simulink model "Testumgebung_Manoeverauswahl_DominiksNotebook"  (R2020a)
settings: Solver=ode4  StartTime=0.0  StopTime=30.0  FixedStep=0.01  RelTol=1e-3
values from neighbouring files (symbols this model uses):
  c = [0;0]    [Testskript_Manoeverauswahl.m]

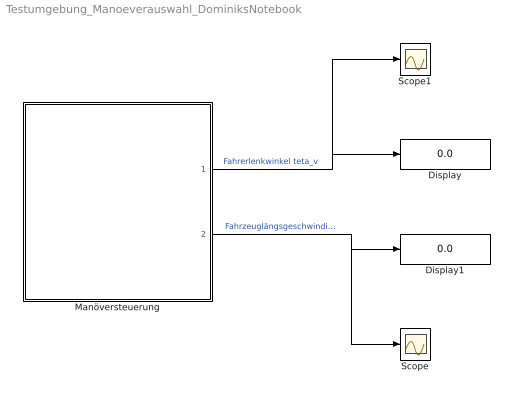
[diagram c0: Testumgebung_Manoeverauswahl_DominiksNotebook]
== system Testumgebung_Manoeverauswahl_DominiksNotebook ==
  Display : Display
  Display1 : Display
  Manöversteuerung : Subsystem
  Scope : Scope
  Scope1 : Scope
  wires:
  Manöversteuerung/2(Fahrzeuglängsgeschwindigkeit KvCx) -> Scope/1, Display1/1  "Fahrzeuglängsgeschwindigkeit KvCx"
  Manöversteuerung/1(Fahrerlenkwinkel teta_v) -> Scope1/1, Display/1  "Fahrerlenkwinkel teta_v"

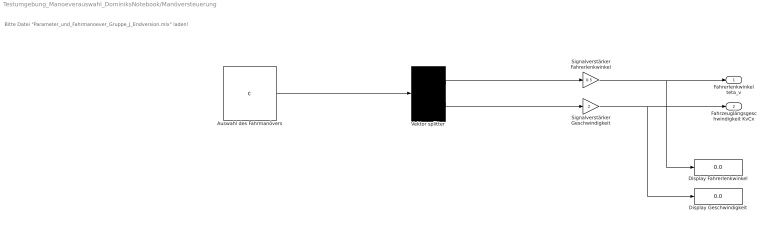
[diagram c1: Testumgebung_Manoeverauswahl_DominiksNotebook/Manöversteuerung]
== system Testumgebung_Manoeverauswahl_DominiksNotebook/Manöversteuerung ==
  note: Bitte Datei "Parameter_und_Fahrmanoever_Gruppe_J_Endversion.mlx" laden!
  Auswahl des Fahrmanövers : Constant  Value=c
  Display Fahrerlenkwinkel : Display
  Display Geschwindigkeit : Display
  Signalverstärker Fahrerlenkwinkel : Gain  Gain=0.5
  Signalverstärker Geschwindigkeit : Gain  Gain=2
  Vektor splitter : Demux  Outputs=2
  Fahrerlenkwinkel teta_v : Outport
  Fahrzeuglängsgeschwindigkeit KvCx : Outport  Port=2
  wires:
  Vektor splitter/1 -> Signalverstärker Fahrerlenkwinkel/1
  Vektor splitter/2 -> Signalverstärker Geschwindigkeit/1
  Signalverstärker Geschwindigkeit/1 -> Fahrzeuglängsgeschwindigkeit KvCx/1, Display Geschwindigkeit/1
  Signalverstärker Fahrerlenkwinkel/1 -> Fahrerlenkwinkel teta_v/1, Display Fahrerlenkwinkel/1
  Auswahl des Fahrmanövers/1 -> Vektor splitter/1
